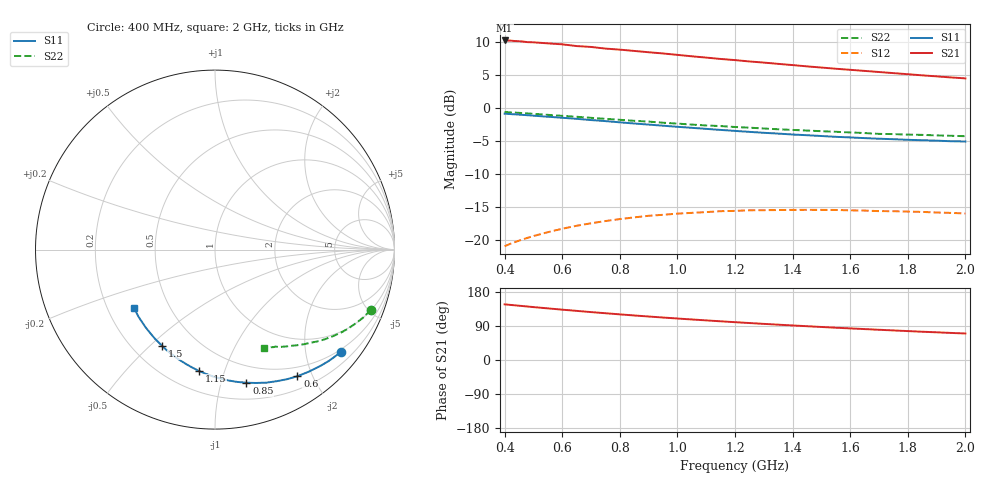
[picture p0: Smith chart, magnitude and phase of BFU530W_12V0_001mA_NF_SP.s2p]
! Filename:  P:\Prog\Test\Noise\ATS_data\Testdata_Net\06 Compressed Noise after Statistics\BFU530W_APM2013_09_A05_12p0V_001mA_NF_CM01_D.sf
! Date/Time: Tue 26/Mar/2013 18:06:02
! BFU530W_APM2013_09_A05_12p0V_1to25mA_NF_CM01_Bias1_R.sf
! Noise Parameter Data File
! BFU530W_APM2013_09_A05_12p0V_1to25mA_NF_CM01
! Date/time: Thu Mar 21 22:54:15 2013
! freq range =  0.4000 to  2.0000 GHz, 37 points
! bias range =  0.9900 to 25.0000 mA, 9 points
! bias supplies used: 1 1 0 0 0 0
! VAR bias_mode= 1  ! Specify V_out, I_out
! VAR bias_var = 1  ! Bias variable = I_out
! VAR V_out= 12.000000
! VAR I_out= 0.990000
! VAR V_in= 0.777400
! VAR I_in= 0.007500
! Device data file deembeded for feedlines and parallel
! Original file: \06 Compressed Noise after Statistics\BFU530W_APM2013_09_A05_12p0V_001mA_NF_CM01_R.sf
! Feed-files: PR019V01_070313_Feed1.s2p, PR019V01_070313_Feed2.s2p
! Parallel-file: PR019V01_070313_Par.s2p
# MHz S MA R 50
!  Freq-MHz  S11-mag  S11-arg  S21-mag  S21-arg  S12-mag  S12-arg  S22-mag  S22-arg
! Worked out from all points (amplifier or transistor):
!   37 points, 400 MHz to 2 GHz, reference 50 ohm
!   highest |S21| = 10.2 dB at 400 MHz (marker M1)
!   |S21| within 3 dB of that: start of sweep to 1.209 GHz
!   unconditionally stable (mu >= 1): nowhere
!   at 500 MHz: K = 0.19, MSG = 14.6 dB, |S12| = -19.3 dB
!   at 1.1 GHz: K = 0.40, MSG = 11.6 dB, |S12| = -15.7 dB
!   at 2 GHz: K = 0.75, MSG = 10.2 dB, |S12| = -15.9 dB
!   lowest NFmin = 0.47 dB at 420 MHz
!   S11 on the Smith chart (normalised r, x): 400 MHz: 0.44, -2.76; 600 MHz: 0.37, -1.79; 850 MHz: 0.34, -1.21; 1.15 GHz: 0.33, -0.82; 1.5 GHz: 0.32, -0.55; 2 GHz: 0.31, -0.29
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400  0.9044 -39.1  3.222 147.0  0.0906 64.8  0.9299 -21.1
420  0.8977 -41.0  3.214 145.4  0.09437 63.8  0.9247 -22.0
460  0.8861 -44.6  3.168 142.6  0.1014 61.6  0.914 -23.8
480  0.8797 -46.3  3.129 141.1  0.1047 60.5  0.9079 -24.7
500  0.873 -48.2  3.119 139.6  0.108 59.5  0.9013 -25.5
600  0.8419 -56.9  3.012 132.8  0.1226 54.7  0.8702 -29.6
650  0.8263 -60.9  2.923 129.7  0.1291 52.5  0.8566 -31.4
700  0.8089 -65.1  2.879 126.4  0.1348 50.4  0.8408 -33.3
750  0.7944 -68.9  2.798 123.4  0.1402 48.4  0.8265 -34.9
800  0.7777 -72.8  2.747 120.5  0.145 46.5  0.8126 -36.6
850  0.7621 -76.7  2.686 117.5  0.1493 44.6  0.7986 -38.1
950  0.7336 -84.0  2.571 112.1  0.1562 41.3  0.7724 -41.2
1050  0.707 -90.8  2.447 107.0  0.1615 38.4  0.7479 -43.8
1150  0.6818 -97.5  2.337 102.1  0.1663 35.6  0.7289 -46.1
1200  0.6701 -100.7  2.291 99.8  0.1672 34.4  0.7171 -47.5
1250  0.6591 -103.8  2.238 97.5  0.1689 33.3  0.7089 -48.5
1350  0.6396 -109.8  2.146 93.2  0.1696 31.3  0.6893 -50.9
1500  0.6132 -118.5  2.013 87.2  0.1701 28.7  0.6668 -54.1
1600  0.5984 -124.1  1.935 83.4  0.1688 27.5  0.6526 -56.2
1750  0.5802 -131.8  1.827 78.1  0.1663 26.3  0.6341 -59.0
1850  0.57 -136.9  1.758 74.6  0.1642 25.6  0.6254 -60.9
2000  0.5579 -144.2  1.668 69.9  0.1598 25.7  0.6113 -63.7
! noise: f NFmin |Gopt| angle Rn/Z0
400  0.4794  0.6848  24.2  0.319
460  0.5374  0.6585  30.03  0.3348
600  0.6136  0.6521  36.46  0.3394
800  0.6678  0.6187  49.43  0.2886
1000  0.7566  0.6364  60.35  0.3176
1200  0.8063  0.6135  72.85  0.2764
1400  0.8817  0.6047  86.23  0.213
1600  0.7757  0.5432  99.33  0.1653
1800  0.9415  0.6175  115.1  0.1357
2000  0.9909  0.6441  124.5  0.1156
